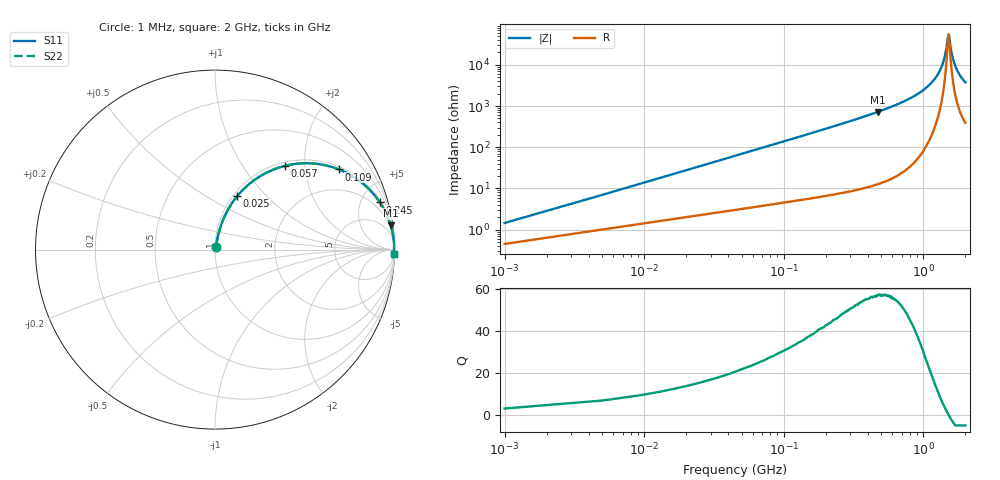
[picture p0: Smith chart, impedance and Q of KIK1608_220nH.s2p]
!version-2
!date-01.2022
!Series
# MHz S RI R 50
!Freq ReS11 ImS11 ReS21 ImS21 ReS12 ImS12 ReS22 ImS22
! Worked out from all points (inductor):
!   501 points, 1 MHz to 2 GHz, reference 50 ohm
!   read as one part in series: L = 220 nH near 9 MHz
!   highest Q = 57.1 at 473 MHz (marker M1), where L = 244 nH
!   self-resonance near 1.513 GHz
!   S11 on the Smith chart (normalised r, x): 1 MHz: 1.01, +0.03; 25 MHz: 1.04, +0.69; 57 MHz: 1.07, +1.58; 109 MHz: 1.10, +3.03; 245 MHz: 1.15, +6.96; 2 GHz: 9, -75
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1  0.00467 0.0137  0.9953 -0.0137  0.9953 -0.0137  0.00467 0.0137
13  0.0458 0.1687  0.9542 -0.1687  0.9542 -0.1687  0.0458 0.1687
25  0.1223 0.2967  0.8777 -0.2967  0.8777 -0.2967  0.1223 0.2967
37  0.2202 0.3885  0.7798 -0.3885  0.7798 -0.3885  0.2202 0.3885
57  0.3888 0.4664  0.6112 -0.4664  0.6112 -0.4664  0.3888 0.4664
109  0.6911 0.4466  0.3089 -0.4466  0.3089 -0.4466  0.6911 0.4466
165  0.8357 0.3579  0.1643 -0.3579  0.1643 -0.3579  0.8357 0.3579
245  0.9189 0.2625  0.0811 -0.2625  0.0811 -0.2625  0.9189 0.2625
337  0.9566 0.1944  0.0434 -0.1944  0.0434 -0.1944  0.9566 0.1944
473  0.979 0.1349  0.021 -0.1349  0.021 -0.1349  0.979 0.1349
669  0.9909 0.0862  0.00914 -0.0862  0.00914 -0.0862  0.9909 0.0862
1003  0.997 0.0403  0.003 -0.0403  0.003 -0.0403  0.997 0.0403
1210  0.9981 0.0216  0.00194 -0.0216  0.00194 -0.0216  0.9981 0.0216
1337  0.9983 0.0119  0.00174 -0.0119  0.00174 -0.0119  0.9983 0.0119
1430  0.9983 0.00562  0.00174 -0.00562  0.00174 -0.00562  0.9983 0.00562
1500  0.9982 0.000969  0.00181 -0.000969  0.00181 -0.000969  0.9982 0.000969
1517  0.9982 -3.31e-05  0.00183 3.31e-05  0.00183 3.31e-05  0.9982 -3.31e-05
1530  0.9982 -0.000777  0.00185 0.000777  0.00185 0.000777  0.9982 -0.000777
1600  0.998 -0.00513  0.00199 0.00513  0.00199 0.00513  0.998 -0.00513
1670  0.9978 -0.00906  0.00216 0.00906  0.00216 0.00906  0.9978 -0.00906
1800  0.9974 -0.0163  0.00259 0.0163  0.00259 0.0163  0.9974 -0.0163
2000  0.9966 -0.0262  0.00343 0.0262  0.00343 0.0262  0.9966 -0.0262
